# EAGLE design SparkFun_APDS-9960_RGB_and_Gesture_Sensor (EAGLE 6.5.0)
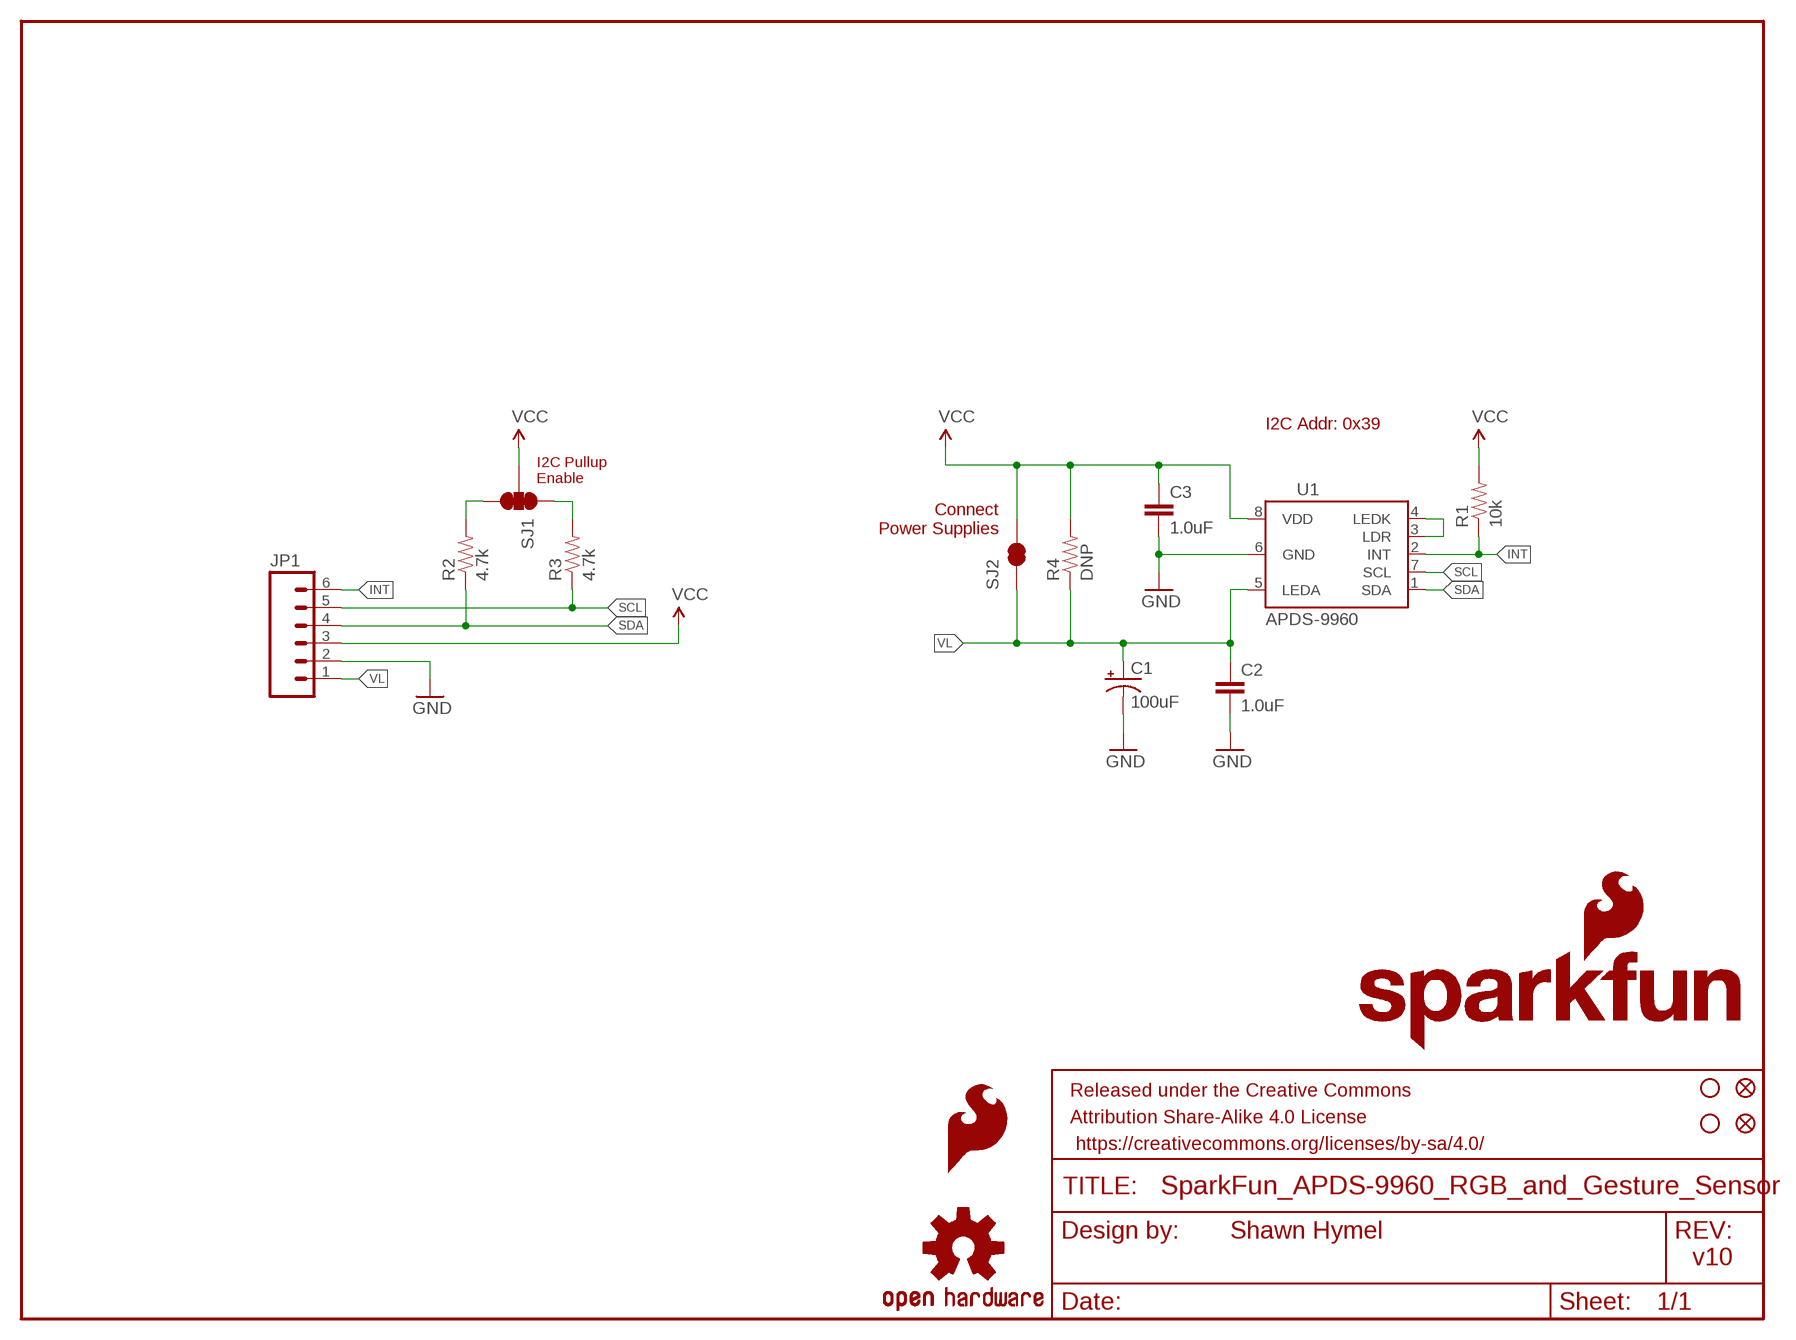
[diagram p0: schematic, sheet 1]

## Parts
C1  100uF  100UF-10V-10%(TANT)  [EIA7343]
C2  1.0uF  1.0UF-16V-10%(0603)  [0603-CAP]
C3  1.0uF  1.0UF-16V-10%(0603)  [0603-CAP]
FID1  FIDUCIAL1X2  [FIDUCIAL-1X2]
FID2  FIDUCIAL1X2  [FIDUCIAL-1X2]
FRAME1  FRAME-LETTER  [CREATIVE_COMMONS]
JP1  M06SIP  [1X06]
LOGO1  SFE_LOGO_FLAME.1_INCH  [SFE_LOGO_FLAME_.1]
LOGO2  OSHW-LOGOS  [OSHW-LOGO-S]
R1  10k  10KOHM1/10W1%(0603)0603  [0603-RES]
R2  4.7k  4.7KOHM1/10W1%(0603)  [0603]
R3  4.7k  4.7KOHM1/10W1%(0603)  [0603]
R4  DNP  RESISTOR0603  [0603-RES]
SJ1  SOLDERJUMPER_2WAYPASTE1&2&3  [SJ_3_PASTE1&2&3]
SJ2  SOLDERJUMPERNC  [SJ_2S]
STANDOFF1  STAND-OFF  [STAND-OFF]
STANDOFF2  STAND-OFF  [STAND-OFF]
U1  APDS-9960  [APDS-9960]
U$1  SFE_LOGO_NAME_FLAME.1_INCH  [SFE_LOGO_NAME_FLAME_.1]

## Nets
GND: C1.C(-) C2.2 C3.2 JP1.2 U1.6(GND)
INT: JP1.6 R1.1 U1.2(INT)
N$1: R2.2 SJ1.3
N$2: R3.2 SJ1.1
N$4: U1.3(LDR) U1.4(LEDK)
SCL: JP1.5 R3.1 U1.7(SCL)
SDA: JP1.4 R2.1 U1.1(SDA)
VCC: C3.1 JP1.3 R1.2 R4.2 SJ1.2 SJ2.2 U1.8(VDD)
VL: C1.A(+) C2.1 JP1.1 R4.1 SJ2.1 U1.5(LEDA)

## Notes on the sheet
- I2C Addr: 0x39
- I2C Pullup
  Enable
- Connect
  Power Supplies
- Shawn Hymel
- v10

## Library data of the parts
C1 = SparkFun-Capacitors:100UF-10V-10%(TANT): CAP-07890; PROD_ID: CAP-07890
C2 C3 = SparkFun-Capacitors:1.0UF-16V-10%(0603): CAP-00868; PROD_ID: CAP-00868
FID1 FID2 = SparkFun-Aesthetics:FIDUCIAL: Fiducial Alignment Points
FRAME1 = SparkFun-Aesthetics:FRAME-LETTER: Schematic Frame
JP1 = SparkFun-Connectors:M06: Header 6 Standard 6-pin 0.1" header. Use with straight break away headers (SKU : PRT-00116), right angle break away headers (PRT-00553), swiss pins (PRT-00743), machine pins (PRT-00117), and female headers (PRT-00115). Molex polarized connector foot print use with SKU : PRT-08094 with associated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
LOGO1 = SparkFun-Aesthetics:SFE_LOGO_FLAME: SFE Logo, flame only
LOGO2 = SparkFun-Aesthetics:OSHW-LOGO: Open Source Hardware Logo This logo indicates the piece of hardware it is found on incorporates a OSHW license and/or adheres to the definition of open source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
R1 = SparkFun-Resistors:10KOHM1/10W1%(0603): RES-00824; PROD_ID: RES-00824; VALUE: 10K
R2 R3 = SparkFun-Resistors:4.7KOHM1/10W1%(0603): RES-07857; PROD_ID: RES-07857
R4 = SparkFun-Resistors:RESISTOR: Resistor
SJ1 = SparkFun-Passives:SOLDERJUMPER_2WAY: Solder Jumper 2 way solder jumper
SJ2 = SparkFun-Retired:SOLDERJUMPER: Solder Jumper
STANDOFF1 STANDOFF2 = SparkFun-Electromechanical:STAND-OFF: #4 Stand Off
U1 = SparkFun-Sensors:APDS-9960: Avago APDS-9960 digital proximity, ambient light, RGB, and gesture sensor.; PROD_ID: SEN-12005
U$1 = SparkFun-Aesthetics:SFE_LOGO_NAME_FLAME: SFE Logo, name and flame

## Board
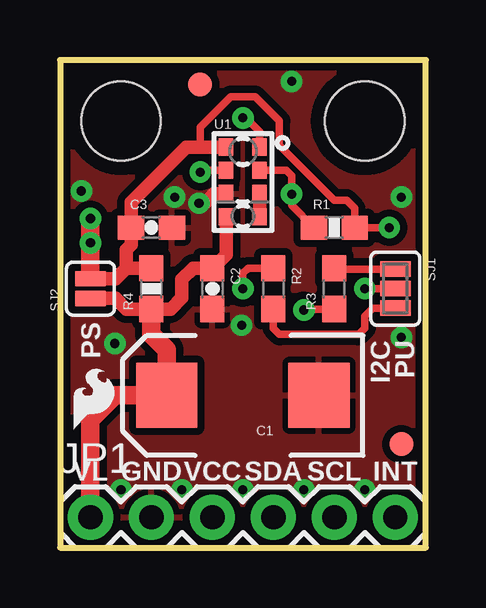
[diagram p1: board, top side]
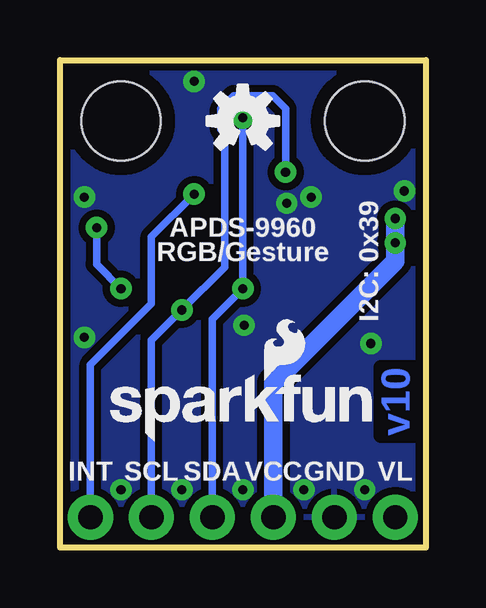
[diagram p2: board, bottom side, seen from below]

Size 15.24 x 20.32 mm. Coordinates in mm from the lower left corner, seen from the top.
Outline: 0,20.32 0,0 15.24,0 15.24,20.32 0,20.32
Copper layers (1*16): Top 0.035mm / dielectric 1.5mm / Bottom 0.035mm
Design rules "SparkFun-2-layer": minimum track width 7mil, minimum drill 15mil, track to track 8mil, track to pad 8mil, pad to pad 8mil, via to via 8mil, smd to smd 8mil, copper to edge 8mil, drill to drill 8mil, minimum pad ring 12mil, minimum via ring 10mil, stop-mask expansion 4mil, vias tented up to drill 20mil, thermal gap 10mil

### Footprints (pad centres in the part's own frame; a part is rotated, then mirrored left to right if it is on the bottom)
EIA7343 = smd 2.55 x 2.7: A 3.17,0; C -3.17,0
0603-CAP = smd 1.1 x 1: 1 -0.85,0; 2 0.85,0
FIDUCIAL-1X2 = smd 1 x 1: 1 0,0
1X06 = drill 1.016 pad 1.88: 1 0,0; 2 2.54,0; 3 5.08,0; 4 7.62,0; 5 10.16,0; 6 12.7,0
0603-RES = smd 1.1 x 1: 1 -0.85,0; 2 0.85,0
0603 = smd 1.1 x 1: 1 -0.85,0; 2 0.85,0
SJ_3_PASTE1&2&3 = smd 0.635 x 1.27: 1 -0.813,0; 2 0,0; 3 0.813,0
SJ_2S = smd 0.635 x 1.27: 1 -0.412,0; 2 0.412,0
STAND-OFF = hole 3.302: 0,0
APDS-9960 = smd 0.6 x 0.72: 1 0.7,1.455; 2 0.7,0.485; 3 0.7,-0.485; 4 0.7,-1.455; 5 -0.7,-1.455; 6 -0.7,-0.485; 7 -0.7,0.485; 8 -0.7,1.455

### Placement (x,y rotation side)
C1  7.62,6.35 180 top
C2  6.35,10.79 270 top
C3  3.81,13.34 0 top
FID1  14.22,4.32 0 top
FID2  5.84,19.3 0 top
FRAME1  not placed on the board
JP1  1.27,1.27 0 top
LOGO1  0.25,4.57 0 top
LOGO2  7.62,17.78 0 bottom
R1  11.43,13.34 0 top
R2  8.89,10.79 270 top
R3  11.43,10.79 90 top
R4  3.81,10.79 90 top
SJ1  13.97,10.79 270 top
SJ2  1.27,10.79 90 top
STANDOFF1  2.54,17.78 0 top
STANDOFF2  12.7,17.78 0 top
U1  7.62,15.24 0 top
U$1  13.59,4.32 0 bottom

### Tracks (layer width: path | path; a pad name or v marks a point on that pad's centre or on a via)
GND  (via drill 0.38)
  Top 0.559: U1.6 6.4,14.76 6.4,14.73 6.07,14.4
  other vias: 5.79,14.35 4.78,14.61 7.57,9.27 7.62,2.41 12.7,2.41 14.22,8.76 10.16,2.41 2.54,2.41 5.08,2.41 2.29,8.51 9.65,19.43 14.22,14.61 0.89,14.86
  pour Top (isolate 0.305): 0,20.32 15.24,20.32 15.24,0 0,0
  pour Bottom (isolate 0.305): 0,20.32 15.24,20.32 15.24,0 0,0
INT  (via drill 0.38)
  Top 0.305: U1.2 9.42,15.72 9.65,15.49 v9.65,14.73 9.65,14.26 R1.1
  Bottom 0.305: JP1.6 13.97,7.62 11.43,10.16 11.43,12.95 v9.65,14.73
N$1
  Top 0.305: R2.2 8.89,9.14 9.14,8.89 12.45,8.89 12.7,9.14 12.7,9.65 13.03,9.98 SJ1.3
N$2
  Top 0.305: SJ1.1 11.47,11.61 R3.2
N$4
  Top 0.559: U1.4 U1.3
SCL  (via drill 0.38)
  Top 0.305: U1.7 5.92,15.72 v5.84,15.65 | R3.1 10.2,9.95 v10.16,9.91
  Bottom 0.305: JP1.5 11.43,8.64 v10.16,9.91 8.38,11.68 8.38,17.27 8.53,17.42 8.53,18.29 8,18.82 6.38,18.82 5.84,18.29 v5.84,15.65
SDA  (via drill 0.38)
  Top 0.305: v7.62,10.79 7.62,11.43 7.83,11.64 R2.1 | U1.1 8.32,17.33 7.75,17.91 v7.62,17.91
  Bottom 0.305: v7.62,17.91 v7.62,10.79 8.89,9.53 JP1.4
VCC  (via drill 0.38)
  Top 0.305: SJ1.2 v12.7,10.79 | v13.72,13.34 R1.2 12.28,14.14 11.94,14.48 11.43,14.48 9.14,16.76 9.14,17.78 8.13,18.8 7.11,18.8 5.84,17.53 5.84,16.7
  Top 0.559: 2.75,11.64 2.32,11.21 SJ2.2 1.27,11.4 | R4.2 2.75,11.64 | 2.75,11.64 2.75,12.41 2.96,12.61 C3.1 2.96,14.39 5.26,16.7 5.84,16.7 U1.8
  Top 0.762: 1.27,11.4 v1.27,12.7 v1.27,13.72
  Bottom 0.305: v13.72,13.34 13.72,11.81 v12.7,10.79
  Bottom 0.762: v1.27,13.72 v1.27,12.7 1.27,11.94 6.35,6.86 JP1.3
VL
  Top 0.559: SJ2.1 2.32,10.38 2.75,9.95 R4.1 4.61,9.95 5.08,10.41 5.08,11.18 5.55,11.64 C2.1 6.92,12.21 U1.5
  Top 0.762: R4.1 3.81,8.89 4.45,8.25 C1.A 2.29,6.35 1.27,5.33 JP1.1

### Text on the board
Bottom: v10
tPlace: PS | I2C | PU | VL | GND | VCC | SDA | SCL | INT
bPlace: APDS-9960 | I2C: 0x39 | RGB/Gesture | VL | GND | VCC | SDA | SCL | INT
tDocu: Shawn Hymel

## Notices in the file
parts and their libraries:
SparkFun-Aesthetics: Licensing: Creative Commons ShareAlike 4.0 International - https://creativecommons.org/licenses/by-sa/4.0
SparkFun-Aesthetics: Released under the Creative Commons Attribution Share-Alike 4.0 License
SparkFun-Aesthetics: https://creativecommons.org/licenses/by-sa/4.0
